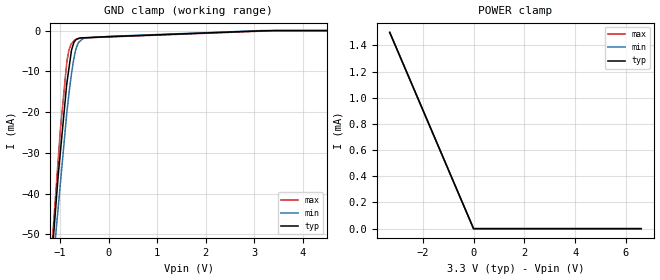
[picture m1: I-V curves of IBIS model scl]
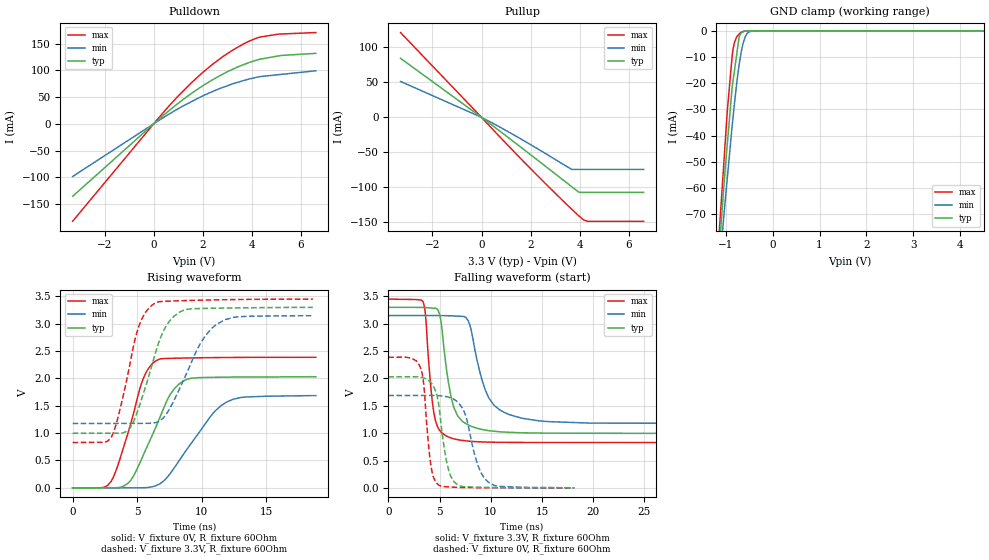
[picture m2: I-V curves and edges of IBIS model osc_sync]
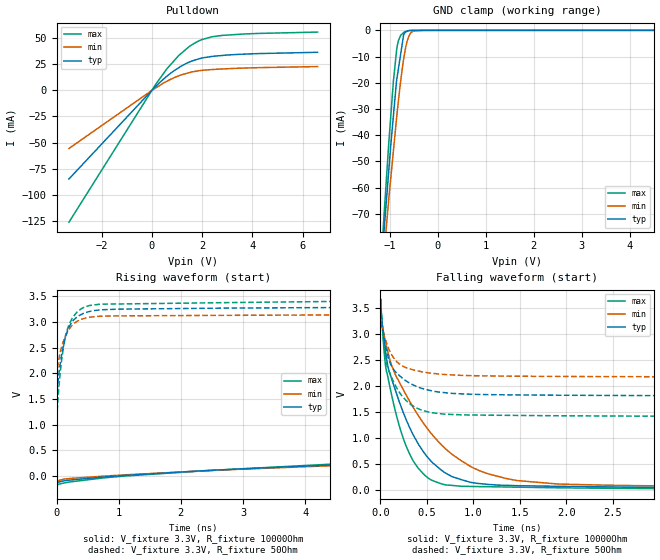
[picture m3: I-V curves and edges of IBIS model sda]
|Texas Instruments Incorporated
| 4-Channel Automotive Digital Amplifiers
| Marketing part#   Digital Voltage Range   Package-type   #pins
| TAS5414CTPHDRQ1   3.15V-3.45V   HTQFP   64
[IBIS Ver]   4.1
[File name]   tas5414c-q1.ibs
[File Rev]   1.0
[Date]   4/23/2013
[Source]
| Texas Instruments Incorporated.
| Analog-eLab Design Center, HPA
| 12500 TI Blvd
| Dallas, TX -75243
[Notes]   Revision History:
| Rev 1.0: 4/23/2013
| - Initial version of the model
| - Model generated from simulations in TISPICE
| - Model matched to SPICE simulation
| - C_comp although listed in numerical order of value are
|   obtained from varying PVT conditions. For PVT conditions for
|   each specific value refer the buffer description under
|   respective [Model]. IBIS model user is responsible for using
|   appropriate C_comp to simulate for Signal Integrity.
| - Model names contains the model for 3.3V [3.15V and 3.45V].
|*   EXCEPTION:   *
|*   - For model scl, there will be leakage currents in GND Clamp IV table   *
|*   because of a pullup resistor (REXT_PU2) is connected to PAD.   *
[Disclaimer]
| This model is designed as an aid for customers of Texas Instruments.
| TI and its licensors and suppliers make no warranties, either expressed
| or implied, with respect to this  model, including the warranties of
| merchantability or fitness for a particular purpose. The model is
| provided solely on an "as is" basis. The entire risk as to its quality
| and performance is with the customer.
[Copyright]
(C) Copyright 2013 Texas Instruments Incorporated.All rights reserved.
|   TAS5414C-Q1PHD
[Component]   TAS5414C-Q1PHD
[Manufacturer]   TI
[Package]   |64 HTQFP  -  PHD package
|   typ   min   max
R_pkg   0.04412   0.03930   0.05048
L_pkg   5.05488nH   4.80826nH   5.42141nH
C_pkg   1.03329pF   1.00463pF   1.05655pF
[Pin]  signal_name   model_name   R_pin   L_pin   C_pin
1   _FAULT   nc   0.03137   4.22518nH  0.97653pF
2   _MUTE   nc   0.02839   3.92421nH  0.96196pF
3   GND   gnd   0.03058   4.03765nH  0.94541pF
4   _STANDBY   nc   0.03481   4.29917nH  0.94913pF
5   D_BYP   nc   0.02492   4.50217nH  1.06967pF
6   _CLIP_OTW   nc   0.05303   5.53068nH  1.05143pF
7   GND   gnd   0.02669   5.85258nH  1.40270pF
8   GND   gnd   0.07184   6.82343nH  1.16318pF
9   GND   gnd   0.07894   7.34695nH  1.18711pF
10   REXT   nc   0.08617   7.92946nH  1.28526pF
11   A_BYP   nc   0.05043   7.46862nH  1.76803pF
12   GND   gnd   0.00681   2.50843nH  0.73690pF
13   IN1_P   nc   0.10597   9.53044nH  1.61760pF
14   GND   gnd   0.00689   2.60547nH  0.77262pF
15   IN2_P   nc   0.11872   10.56253nH 1.90955pF
16   GND   gnd   0.00663   2.72598nH  0.78981pF
17   GND   gnd   0.00659   2.71972nH  0.79074pF
18   IN_M   nc   0.03668   10.50914nH 16.41059pF
19   IN3_P   nc   0.10631   9.60120nH  9.29902pF
20   IN4_P   nc   0.09975   9.07404nH  3.64723pF
21   GND   gnd   0.00682   2.51052nH  0.73501pF
22   GND   gnd   0.09029   8.28010nH  1.37376pF
23   GND   gnd   0.08492   7.84104nH  1.79616pF
24   GND   gnd   0.07970   7.40699nH  1.33473pF
25   GND   gnd   0.07481   7.04661nH  1.35491pF
26   GND   gnd   0.00660   2.40427nH  0.70816pF
27   PVDD   power   0.02737   6.24103nH  1.53724pF
28   PVDD   power   0.02471   5.69064nH  1.63098pF
29   PVDD   power   0.02119   5.25315nH  1.42708pF
30   GND   gnd   0.02568   4.77009nH  1.29295pF
31   GND   gnd   0.02312   4.22107nH  1.28427pF
32   GND   gnd   0.00661   2.72247nH  0.79031pF
33   OUT4_P   nc   0.01604   5.09325nH  2.43311pF
34   OUT4_M   nc   0.01809   5.36607nH  2.60484pF
35   GND   gnd   0.02686   5.12703nH  1.24608pF
36   OUT3_P   nc   0.01859   5.48658nH  2.06803pF
37   OUT3_M   nc   0.02169   5.99495nH  2.64685pF
38   GND   gnd   0.06641   6.50464nH  1.36354pF
39   GND   gnd   0.07045   6.75928nH  1.36985pF
40   CP_BOT   nc   0.07386   6.96310nH  1.32704pF
41   CP   nc   0.07840   7.29730nH  1.39365pF
42   CPC_TOP   nc   0.08329   7.70383nH  1.66684pF
43   GND   gnd   0.04867   7.39306nH  2.36940pF
44   OUT2_P   nc   0.02847   9.17504nH  93.73744pF
45   OUT2_M   nc   0.03204   9.85413nH  121.16052pF
46   GND   gnd   0.06141   9.07455nH  22.01920pF
47   OUT1_P   nc   0.03478   11.37525nH 8.77088pF
48   OUT1_M   nc   0.03824   13.32382nH 4.94813pF
49   GND   gnd   0.00679   2.75402nH  0.78526pF
50   GND   gnd   0.06623   9.62334nH  2.30930pF
51   GND   gnd   0.06217   9.10112nH  2.12088pF
52   PVDD   power   0.04150   10.49268nH 2.19882pF
53   PVDD   power   0.03825   8.08597nH  2.40014pF
54   PVDD   power   0.03446   7.38172nH  2.19651pF
55   GND   gnd   0.00670   2.41379nH  0.71307pF
56   GND   gnd   0.07948   7.37443nH  1.19311pF
57   GND   gnd   0.07424   6.98767nH  1.18519pF
58   GND   gnd   0.06924   6.66542nH  1.16031pF
59   GND   gnd   0.06433   6.34416nH  1.13516pF
60   GND   gnd   0.05967   6.04702nH  1.10459pF
61   OSC_SYNC   osc_sync   0.05048   5.42141nH  1.05655pF
62   I2C_ADDR   nc   0.04649   5.17321nH  1.05134pF
63   SDA   sda   0.04257   4.93498nH  1.03870pF
64   SCL   scl   0.03930   4.80826nH  1.00463pF
| Models and submodels in the file (3): scl (Input), osc_sync (I/O), sda (I/O_open_drain)
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|   scl Model
[Model]   scl
Model_type   Input
Vinl = 1.1
Vinh = 2.1
|   typ   min   max
|   (nom PVT)   (fast PVT)   (slow PVT)
C_comp   2.371e-12   2.118e-12   2.507e-12
| Where nom  PVT is Nominal Process, 3.3V, 27C
|   Fast PVT is Strong Process,  3.45V, -40C
|   Slow PVT is Weak Process,   3.15V, 105C
[Voltage Range]   3.3   3.15   3.45
|Junction Temperature
[Temperature Range]   27   105   -40
[Power Clamp Reference]   3.3   3.15   3.45
[GND Clamp Reference]   0   0   0
[GND Clamp]
|   Voltage   I(typ)   I(min)   I(max)
-3.3V     -528.8mA   -490.8mA   -581.5mA
-1.17V    -55.98mA   -60.8mA    -53.73mA
-1.036V   -35.46mA   -43.33mA   -31.6mA
-993.6mV  -30.03mA   -37.75mA   -24.54mA
-859mV    -12.98mA   -20.14mA   -7.662mA
-817.6mV  -9.475mA   -15.77mA   -4.863mA
-762.3mV  -4.791mA   -10.52mA   -3.199mA
-652.1mV  -2.116mA   -3.837mA   -2.056mA
-510.3mV  -1.761mA   -1.85mA    -1.819mA
-3.15mV   -1.501mA   -1.433mA   -1.57mA
3.147V    -75.67uA   -1.431uA   -137.8uA
6.6V      0A         0A         0A
[POWER Clamp]
|   Voltage   I(typ)   I(min)   I(max)
-3.3V     1.5mA      1.5mA      1.5mA
-2.296V   1.044mA    1.044mA    1.044mA
-39.41fV  0A         0A         0A
6.6V      0A         0A         0A
|   osc_sync Model
[Model]   osc_sync
Model_type   I/O
Polarity   Inverting
Enable   Active-High
Vinl = 0.8
Vinh = 2
Vmeas = 1.65
Vref = 0
Cref = 75pF
Rref = 60
|   typ   min   max
|   (nom PVT)   (fast PVT)   (slow PVT)
C_comp   3.261e-12   2.889e-12   3.532e-12
| Where nom  PVT is Nominal Process, 3.3V, 27C
|   Fast PVT is Strong Process,  3.45V, -40C
|   Slow PVT is Weak Process,   3.15V, 105C
[Voltage Range]   3.3   3.15   3.45
|Junction Temperature
[Temperature Range]   27   105   -40
[Pullup Reference]   3.3   3.15   3.45
[Pulldown Reference]   0   0   0
[Power Clamp Reference]   3.3   3.15   3.45
[GND Clamp Reference]   0   0   0
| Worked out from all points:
|   slope of the pulldown table from 0 to 0.495 V, typ, clamps not added: 25.1 ohm
|   slope of the pullup table from 0 to 0.495 V, typ, clamps not added: 37.8 ohm
|   GND clamp passes 1 mA (typ) near -0.68 V on its own axis
|   falling waveform, V_fixture 3.3V, R_fixture 60Ohm: 20-80 % time 1.15ns typ, 1.86ns min, 743ps max; typ from 3.3 V to 0.996 V
|   rising waveform, V_fixture 0V, R_fixture 60Ohm: 20-80 % time 2.25ns typ, 3.04ns min, 1.74ns max; typ from 0 V to 2.03 V
|   rising waveform, V_fixture 3.3V, R_fixture 60Ohm: 20-80 % time 1.86ns typ, 2.4ns min, 1.5ns max; typ from 0.997 V to 3.3 V
|   falling waveform, V_fixture 0V, R_fixture 60Ohm: 20-80 % time 963ps typ, 1.41ns min, 660ps max; typ from 2.03 V to 0 V
[Pulldown]
|   Voltage   I(typ)   I(min)   I(max)
-3.3V     -135.6mA   -98.45mA   -182.3mA
607.2mV   24.05mA    17.65mA    32.52mA
1.49V     55.3mA     40.34mA    74.74mA
2.374V    81.76mA    59.89mA    110.4mA
3.222V    102.2mA    74.91mA    138mA
3.812V    113.4mA    82.94mA    153mA
4.309V    120.7mA    88.25mA    162.1mA
5.188V    127.9mA    92.47mA    168mA
6.6V      131.8mA    99.22mA    170.7mA
[GND Clamp]
|   Voltage   I(typ)   I(min)   I(max)
-3.3V     -761.3mA   -689.3mA   -866.8mA
-1.128V   -81.2mA    -89.74mA   -74.56mA
-1.033V   -58.29mA   -69.49mA   -48.93mA
-966mV    -43.52mA   -56.5mA    -30.79mA
-859mV    -21.17mA   -35.84mA   -9.104mA
-769.3mV  -9.598mA   -20.87mA   -2.399mA
-712.8mV  -2.303mA   -12.92mA   -1.232mA
-686.5mV  -1.366mA   -10.01mA   -708.3uA
-626.9mV  -363.7uA   -4.661mA   -273uA
-541.8mV  -39.53uA   -977.3uA   -47.82uA
-302.4mV  -2.582uA   -2.001uA   -60.65nA
6.6V      0A         0A         0A
[Pullup]
|   Voltage   I(typ)   I(min)   I(max)
-3.3V     84.47mA    51.38mA    121.3mA
0V        0A         0A         0A
1.784V    -47.73mA   -34.72mA   -65.86mA
3.67V     -99.28mA   -74.48mA   -131.5mA
3.947V    -106.7mA   -74.51mA   -140.6mA
4.14V     -107.4mA   -74.51mA   -146.4mA
4.309V    -107.4mA   -74.51mA   -148.8mA
6.6V      -107.4mA   -74.51mA   -148.8mA
[POWER Clamp]
|   Voltage   I(typ)   I(min)   I(max)
-3.3V     0A         0A         0A
0V        0A         0A         0A
6.6V      0A         0A         0A
[Ramp]
R_load = 60
|   typ   min   max
dV/dt_r   1.21806/2.25181e-09   1.01313/3.04493e-09   1.43224/1.74063e-09
dV/dt_f   1.38213/1.1498e-09   1.18398/1.83615e-09   1.57291/7.41541e-10
[Falling Waveform]
V_fixture = 3.3V
V_fixture_min = 3.15V
V_fixture_max = 3.45V
R_fixture = 60Ohm
|   Time   V(typ)   V(min)   V(max)
0s        3.3V       3.15V      3.45V
3.395ns   3.297V     3.15V      3.402V
4.2ns     3.287V     3.15V      1.737V
4.555ns   3.283V     3.15V      1.265V
5.08ns    3.107V     3.149V     1.034V
6.135ns   1.655V     3.145V     911.2mV
7.805ns   1.15V      3.054V     854.6mV
9.47ns    1.057V     1.785V     837.7mV
11.85ns   1.015V     1.336V     831.1mV
37ns      996.5mV    1.177V     828.5mV
[Rising Waveform]
V_fixture = 0V
V_fixture_min = 0V
V_fixture_max = 0V
R_fixture = 60Ohm
|   Time   V(typ)   V(min)   V(max)
0s        906.9fV    65.46pV    5.326fV
2.99ns    899.5uV    217.2uV    122.3mV
4.51ns    142.2mV    531.5uV    1.182V
5.47ns    596.8mV    2.602mV    1.996V
6.44ns    1.11V      39.94mV    2.321V
7.525ns   1.694V     253.4mV    2.365V
8.305ns   1.911V     518.6mV    2.37V
10.86ns   2.019V     1.358V     2.379V
11.94ns   2.022V     1.57V      2.381V
18.82ns   2.028V     1.684V     2.385V
[Rising Waveform]
V_fixture = 3.3V
V_fixture_min = 3.15V
V_fixture_max = 3.45V
R_fixture = 60Ohm
|   Time   V(typ)   V(min)   V(max)
0s        996.6mV    1.177V     828.7mV
3ns       997.3mV    1.177V     927.6mV
4.52ns    1.122V     1.177V     2.365V
5.27ns    1.569V     1.177V     3.038V
6.225ns   2.313V     1.184V     3.351V
6.995ns   2.848V     1.271V     3.406V
7.855ns   3.138V     1.601V     3.414V
9.905ns   3.276V     2.644V     3.428V
11.24ns   3.282V     3.002V     3.435V
18.59ns   3.296V     3.145V     3.447V
[Falling Waveform]
V_fixture = 0V
V_fixture_min = 0V
V_fixture_max = 0V
R_fixture = 60Ohm
|   Time   V(typ)   V(min)   V(max)
0s        2.03V      1.689V     2.387V
3.12ns    2.023V     1.69V      2.2V
3.455ns   2.008V     1.69V      1.892V
4.135ns   1.928V     1.69V      432.6mV
4.88ns    1.565V     1.686V     56.07mV
5.68ns    484.3mV    1.667V     19.91mV
6.765ns   56.65mV    1.568V     9.49mV
8.71ns    12.48mV    428mV      2.928mV
9.765ns   7.776mV    103.9mV    1.627mV
18.15ns   315.5uV    2.22mV     164uV
|   sda Model
[Model]   sda
Model_type   I/O_open_drain
Polarity   Inverting
Vinl  = 1.1
Vinh = 2.1
Vmeas = 1.65
Vref = 3.3
Cref = 400pF
Rref = 10000
|   typ   min   max
|   (nom PVT)   (fast PVT)   (slow PVT)
C_comp   3.144e-12   2.914e-12   3.281e-12
| Where nom  PVT is Nominal Process, 3.3V, 27C
|   Fast PVT is Strong Process,  3.45V, -40C
|   Slow PVT is Weak Process,   3.15V, 105C
[Voltage Range]   3.3   3.15   3.45
|Junction Temperature
[Temperature Range]   27   105   -40
[Pullup Reference]   3.3   3.15   3.45
[Pulldown Reference]   0   0   0
[Power Clamp Reference]   3.3   3.15   3.45
[GND Clamp Reference]   0   0   0
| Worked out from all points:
|   slope of the pulldown table from 0 to 0.495 V, typ, clamps not added: 42.9 ohm
|   GND clamp passes 1 mA (typ) near -0.69 V on its own axis
|   falling waveform, V_fixture 3.3V, R_fixture 10000Ohm: 20-80 % time 429ps typ, 699ps min, 276ps max; typ from 3.3 V to 0.013 V
|   rising waveform, V_fixture 3.3V, R_fixture 10000Ohm: 20-80 % time 88.7ns typ, 94.9ns min, 83.5ns max; typ from 0.013 V to 3.29 V
|   falling waveform, V_fixture 3.3V, R_fixture 50Ohm: 20-80 % time 239ps typ, 220ps min, 202ps max; typ from 3.3 V to 1.8 V
|   rising waveform, V_fixture 3.3V, R_fixture 50Ohm: 20-80 % time 200ps typ, 212ps min, 194ps max; typ from 1.8 V to 3.3 V
[Pulldown]
|   Voltage   I(typ)   I(min)   I(max)
-3.3V     -85.04mA   -55.74mA   -126.5mA
186.3mV   4.618mA    2.877mA    6.983mA
607.2mV   13.84mA    8.991mA    21.02mA
1.073V    21.83mA    14.09mA    33.62mA
1.49V     27.25mA    17.1mA     42.18mA
1.966V    30.95mA    19.21mA    48.66mA
2.374V    32.61mA    20.03mA    51.46mA
2.815V    33.65mA    20.66mA    52.92mA
4.14V     35.33mA    21.84mA    54.69mA
6.6V      36.67mA    22.95mA    56.08mA
[GND Clamp]
|   Voltage   I(typ)   I(min)   I(max)
-3.3V     -729.8mA   -668.1mA   -819.8mA
-1.135V   -79.69mA   -87.85mA   -74.46mA
-1.028V   -54.76mA   -65.54mA   -44.41mA
-928.1mV  -33.02mA   -46.34mA   -19.71mA
-859mV    -19.07mA   -33.25mA   -7.478mA
-776.2mV  -9.2mA     -19.63mA   -1.942mA
-712.8mV  -1.634mA   -10.92mA   -853.5uA
-696.9mV  -1.199mA   -9.219mA   -590.2uA
-639.4mV  -346.4uA   -4.099mA   -302.6uA
-560.7mV  -40.41uA   -899uA     -37.12uA
-311.9mV  -17.31uA   -2.134uA   -51.41nA
6.6V      0A         0A         0A
[POWER Clamp]
|   Voltage   I(typ)   I(min)   I(max)
-3.3V     0A         0A         0A
0V        0A         0A         0A
6.6V      0A         0A         0A
[Ramp]
R_load = 10000
|   typ   min   max
dV/dt_r   1.96904/8.86641e-08   1.87439/9.48039e-08   2.06225/8.34121e-08
dV/dt_f   1.97232/4.29187e-10   1.87886/6.98769e-10   2.06466/2.76047e-10
[Falling Waveform]
V_fixture = 3.3V
V_fixture_min = 3.15V
V_fixture_max = 3.45V
R_fixture = 10000Ohm
|   Time   V(typ)   V(min)   V(max)
0s        3.3V       3.15V      3.45V
5ps       3.518V     3.345V     3.679V
40ps      2.91V      2.985V     2.697V
65ps      2.571V     2.785V     2.298V
265ps     1.409V     1.87V      900.7mV
460ps     740.4mV    1.292V     310.8mV
715ps     305.1mV    766.3mV    88.78mV
1.15ns    102.3mV    310.8mV    56.68mV
1.92ns    63.88mV    107.3mV    35.14mV
14.34ns   12.61mV    20.29mV    8.946mV
[Rising Waveform]
V_fixture = 3.3V
V_fixture_min = 3.15V
V_fixture_max = 3.45V
R_fixture = 10000Ohm
|   Time   V(typ)   V(min)   V(max)
0s        12.8mV     18.56mV    8.9mV
5ps       -183.4mV   -123.1mV   -258.1mV
250ps     -76.51mV   -46.77mV   -111.8mV
2.345ns   100.6mV    98.77mV    97.7mV
16.55ns   781mV      665.9mV    925.5mV
42.28ns   1.619V     1.438V     1.801V
75.22ns   2.281V     2.08V      2.481V
113.6ns   2.743V     2.544V     2.937V
213.4ns   3.187V     3.017V     3.355V
400ns     3.295V     3.143V     3.446V
[Falling Waveform]
V_fixture = 3.3V
V_fixture_min = 3.15V
V_fixture_max = 3.45V
R_fixture = 50Ohm
|   Time   V(typ)   V(min)   V(max)
0s        3.3V       3.15V      3.45V
5ps       3.506V     3.335V     3.658V
15ps      3.275V     3.202V     3.319V
35ps      3.006V     3.023V     2.885V
70ps      2.668V     2.814V     2.415V
110ps     2.426V     2.647V     2.215V
180ps     2.25V      2.465V     1.952V
375ps     2.003V     2.301V     1.592V
635ps     1.883V     2.231V     1.468V
10.47ns   1.803V     2.168V     1.413V
[Rising Waveform]
V_fixture = 3.3V
V_fixture_min = 3.15V
V_fixture_max = 3.45V
R_fixture = 50Ohm
|   Time   V(typ)   V(min)   V(max)
0s        1.802V     2.166V     1.412V
5ps       1.486V     1.978V     1.024V
10ps      1.615V     2.029V     1.241V
25ps      1.857V     2.19V      1.54V
80ps      2.347V     2.507V     2.236V
135ps     2.662V     2.705V     2.674V
200ps     2.897V     2.858V     2.946V
395ps     3.148V     3.054V     3.257V
705ps     3.238V     3.115V     3.349V
35.78ns   3.3V       3.15V      3.45V
